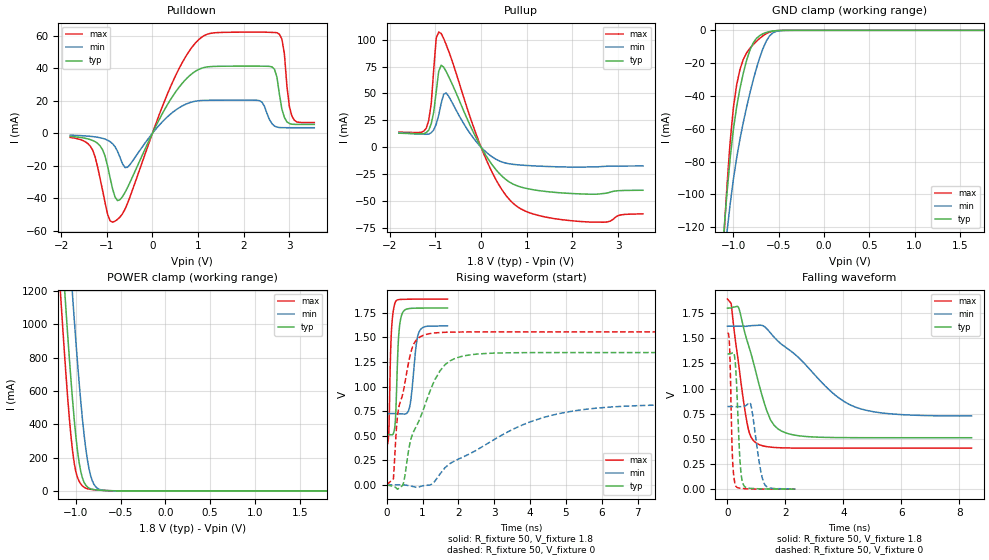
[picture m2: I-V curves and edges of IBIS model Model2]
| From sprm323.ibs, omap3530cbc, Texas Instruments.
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| Model based on original model for BQ0232CS_7LM
|   Sub model 0232CS_PD_PU_OFF_1P8
[model]   Model2
|[Input Load]   PI
|[Output Drive]
|Voltage   1.8V
|Mode   I/O
Model_type   I/O
Polarity   Non-Inverting
Enable   Active-Low
Vinl =  0.63
Vinh =  1.17
Cref =  15.0000pF
Rref =  100.0000M
Vref =  0V
Vmeas =  0.9
C_comp   0.8836195p   0.7578727p   1.042532p
[Model Spec]
Vinl   0.63   0.567   0.6615
Vinh   1.17   1.053   1.2285
[Temperature Range]   25   125   -40
[Voltage Range]   1.8   1.62   1.89
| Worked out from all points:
|   slope of the pulldown table from 0 to 0.27 V, typ, clamps not added: 18.2 ohm
|   slope of the pullup table from 0 to 0.27 V, typ, clamps not added: 15.1 ohm
|   GND clamp passes 1 mA (typ) near -0.62 V on its own axis
|   POWER clamp passes 1 mA (typ) near -0.57 V on its own axis
|   rising waveform, R_fixture 50, V_fixture 1.8: 20-80 % time 82.3ps typ, 143ps min, 65.7ps max; typ from 0.511 V to 1.8 V
|   rising waveform, R_fixture 50, V_fixture 0: 20-80 % time 779ps typ, 2.51ns min, 383ps max; typ from 0 V to 1.35 V
|   falling waveform, R_fixture 50, V_fixture 1.8: 20-80 % time 759ps typ, 1.98ns min, 424ps max; typ from 1.8 V to 0.511 V
|   falling waveform, R_fixture 50, V_fixture 0: 20-80 % time 127ps typ, 250ps min, 81.7ps max; typ from 1.35 V to 0.001 V
[POWER_clamp]
-1.8V     7.03A      7.477A     6.772A
-1.182V   1.672A     2.34A      1.267A
-1.164V   1.518A     2.189A     1.114A
-1.127V   1.216A     1.889A     820.4mA
-1.073V   791.2mA    1.448A     431.2mA
-1.036V   538.2mA    1.164A     234.5mA
-963.6mV  168.9mA    647.7mA    57.17mA
-909.1mV  51.94mA    338.6mA    22mA
-872.7mV  24.12mA    189.8mA    13.24mA
-818.2mV  9.796mA    62.59mA    8.394mA
-709.1mV  3.779mA    4.968mA    3.659mA
1.8V      5.391nA    3.441nA    8.971nA
[Pulldown]
-1.8V     -1.896mA   -1.14mA    -2.549mA
-1.364V   -3.858mA   -1.868mA   -7.811mA
-1.145V   -7.758mA   -2.749mA   -27.9mA
-818.2mV  -39.37mA   -8.28mA    -54.21mA
-545.5mV  -33.5mA    -20.95mA   -43.25mA
654.5mV   30.89mA    16.9mA     43.69mA
1.418V    41.32mA    20.41mA    62.11mA
2.345V    41.43mA    20.12mA    62.44mA
2.618V    40.99mA    5.968mA    62.24mA
2.782V    24.07mA    3.525mA    61.09mA
3.055V    5.586mA    3.449mA    10.68mA
3.545V    5.467mA    3.446mA    6.63mA
[Pullup]
-1.8V     13mA       13.47mA    13.94mA
-1.2V     13.58mA    11.97mA    17.52mA
-1.091V   21.69mA    13.4mA     40.44mA
-1.036V   32.56mA    16.02mA    72.05mA
-981.8mV  51.54mA    21.35mA    101.5mA
-927.3mV  70.65mA    29.72mA    107.1mA
-818.2mV  74.4mA     49.19mA    101mA
-763.6mV  70.3mA     50.34mA    95.36mA
54.55mV   -4.056mA   -2.362mA   -5.695mA
709.1mV   -34.52mA   -16.04mA   -52.48mA
2.127V    -43.43mA   -18.65mA   -69.01mA
3.545V    -40.12mA   -17.52mA   -62.13mA
[GND_clamp]
-1.8V     -750.6mA   -623.3mA   -941.3mA
-1.109V   -125.7mA   -143.5mA   -129.8mA
-1.073V   -100.3mA   -123.9mA   -96.46mA
-1.036V   -78.28mA   -106.2mA   -68.22mA
-1V       -60.33mA   -90.75mA   -47.08mA
-963.6mV  -46.48mA   -77.6mA    -33.12mA
-890.9mV  -26.13mA   -56.16mA   -17.76mA
-818.2mV  -12.14mA   -38.32mA   -10.94mA
-709.1mV  -3.177mA   -16.6mA    -4.873mA
-600mV    -740.6uA   -3.353mA   -1.096mA
-490.9mV  -93.6uA    -272.6uA   -80.84uA
1.764V    4.431nA    31.01nA    4.817nA
[Ramp]
dV/dt_f  0.7838235/0.7675472n  0.5431734/2.017101n   0.9061631/0.4292738n
dV/dt_r   0.834573/0.7801827n  0.5086842/2.534977n   0.9673336/0.383387n
R_load = 50
[Rising Waveform]
R_fixture = 50
V_fixture = 1.8
V_fixture_min = 1.62
V_fixture_max = 1.89
0s        511.5mV    724.7mV    407.9mV
60ps      511.3mV    724.7mV    531.3mV
108ps     510mV      724.8mV    1.321V
136ps     508.7mV    724.9mV    1.578V
236ps     618.3mV    724.9mV    1.854V
338ps     1.532V     723.9mV    1.885V
436ps     1.745V     721.3mV    1.887V
656ps     1.795V     818.7mV    1.889V
900ps     1.798V     1.553V     1.889V
1.696ns   1.799V     1.617V     1.89V
[Rising Waveform]
R_fixture = 50
V_fixture = 0
V_fixture_min = 0
V_fixture_max = 0
0s        196.3nV    87.52nV    426.7nV
188ps     -15.38mV   13.6uV     60.9mV
310ps     -44.06mV   178.9uV    719.3mV
450ps     -643.9uV   -16.79uV   926.1mV
720ps     514.3mV    -15.78mV   1.402V
980ps     722.8mV    -11.93mV   1.514V
1.49ns    1.161V     111.4mV    1.55V
2.18ns    1.314V     291.6mV    1.555V
5.068ns   1.346V     742.9mV    1.556V
9.856ns   1.346V     818.1mV    1.556V
[Falling Waveform]
R_fixture = 50
V_fixture = 1.8
V_fixture_min = 1.62
V_fixture_max = 1.89
0s        1.8V       1.62V      1.89V
126ps     1.801V     1.62V      1.847V
364ps     1.814V     1.62V      1.29V
680ps     1.473V     1.62V      651.8mV
1.004ns   1.135V     1.628V     456.9mV
1.488ns   687.2mV    1.551V     417.9mV
2.108ns   550.7mV    1.39V      409.6mV
3.598ns   513.8mV    964mV      407.9mV
4.418ns   512mV      815.3mV    407.9mV
8.418ns   511.5mV    727.9mV    407.9mV
[Falling Waveform]
R_fixture = 50
V_fixture = 0
V_fixture_min = 0
V_fixture_max = 0
0s        1.346V     821.4mV    1.556V
74ps      1.346V     821.5mV    1.405V
184ps     1.358V     820.9mV    248.4mV
274ps     1.241V     820.5mV    39.55mV
432ps     279.9mV    820.2mV    10.31mV
540ps     50.55mV    821.8mV    6.912mV
794ps     8.036mV    850.4mV    2.21mV
1.12ns    3.398mV    224.3mV    1.168mV
1.304ns   2.173mV    37.02mV    775.2uV
2.342ns   692.6uV    3.25mV     84.03uV
